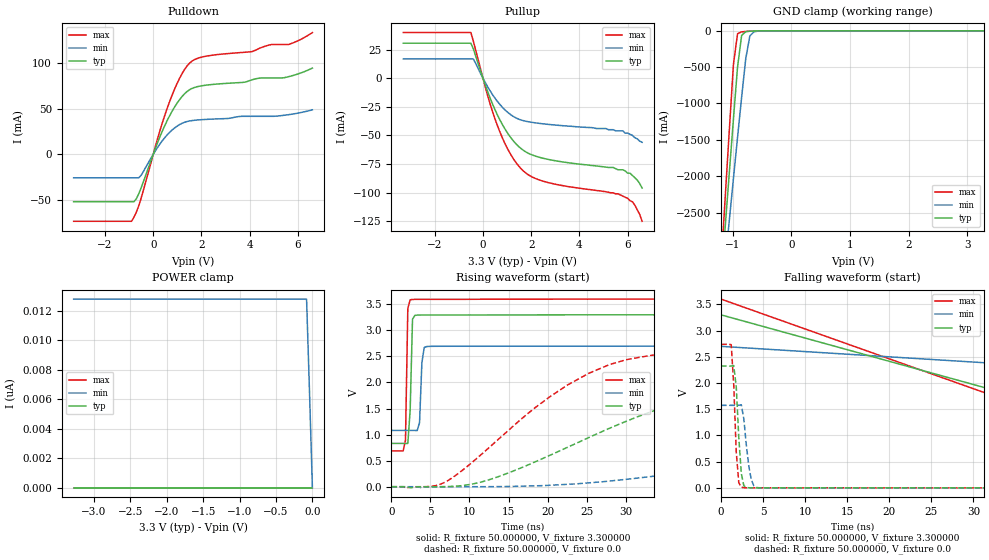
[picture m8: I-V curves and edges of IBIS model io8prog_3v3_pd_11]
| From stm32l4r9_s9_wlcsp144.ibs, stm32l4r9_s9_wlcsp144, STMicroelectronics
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|   Model io8prog_3v3_pd_11
[Model]  io8prog_3v3_pd_11
Model_type I/O
Polarity   Non-Inverting
Enable   Active-Low
Vinl =   0.990000V
Vinh =   2.310000V
Vmeas =  1.650000V
Cref =   100.000000nF
Rref =   1.000000k
Vref =   3.300000V
C_comp   2.267200pF   2.233100pF   2.322300pF
[Temperature Range]   25.000000   0.125000k   -40.000000
[Pullup Reference]   3.300000V   2.700000V   3.600000V
[Pulldown Reference]   0.0V   0.0V   0.0V
[POWER Clamp Reference]   3.300000V   2.700000V   3.600000V
[GND Clamp Reference]   0.0V   0.0V   0.0V
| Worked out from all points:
|   slope of the pulldown table from 0 to 0.495 V, typ, clamps not added: 15.3 ohm
|   slope of the pullup table from 0 to 0.495 V, typ, clamps not added: 18.1 ohm
|   GND clamp passes 1 mA (typ) near -0.58 V on its own axis
|   rising waveform, R_fixture 50.000000, V_fixture 3.300000: 20-80 % time 299ps typ, 253ps min, 207ps max; typ from 0.831 V to 3.3 V
|   rising waveform, R_fixture 50.000000, V_fixture 0.0: 20-80 % time 24.3ns typ, 50.8ns min, 14.5ns max; typ from 0 V to 2.32 V
|   falling waveform, R_fixture 50.000000, V_fixture 3.300000: 20-80 % time 33.4ns typ, 61.6ns min, 30.7ns max; typ from 3.3 V to 0.831 V
|   falling waveform, R_fixture 50.000000, V_fixture 0.0: 20-80 % time 498ps typ, 673ps min, 456ps max; typ from 2.32 V to 0 V
[Pulldown]
|Voltage   I(typ)   I(min)   I(max)
-3.3V     -51.86mA   -25.67mA   -73.32mA
-900mV    -51.86mA   -25.67mA   -73.32mA
-700mV    -48.68mA   -25.67mA   -63.27mA
-500mV    -36.68mA   -22.92mA   -47.9mA
200mV     14.09mA    8.363mA    18.97mA
700mV     43.2mA     24.54mA    59.15mA
1.2V      63.38mA    34mA       88.53mA
1.6V      72.01mA    36.89mA    101.8mA
4.1V      81.58mA    41.61mA    112.4mA
4.9V      83.61mA    41.61mA    120.1mA
5.6V      84.89mA    43.33mA    120.1mA
6.6V      94.39mA    48.68mA    133.3mA
[Pullup]
|Voltage   I(typ)   I(min)   I(max)
-3.3V     30.51mA    16.73mA    39.79mA
-500mV    30.51mA    16.73mA    39.79mA
-400mV    25.73mA    16.73mA    32.44mA
200mV     -11.99mA   -7.69mA    -15.6mA
500mV     -27.53mA   -17.49mA   -35.6mA
1V        -47.29mA   -29.38mA   -60.81mA
1.5V      -60.05mA   -35.95mA   -77.15mA
1.9V      -65.77mA   -38.13mA   -84.64mA
2.6V      -70.47mA   -40.14mA   -90.6mA
5.6V      -80mA      -46mA      -101mA
6.2V      -85mA      -50mA      -108mA
6.6V      -96mA      -56mA      -125mA
[GND_clamp]
|Voltage   I(typ)   I(min)   I(max)
-3.3V     -9.456A    -9.706A    -9.779A
-1.2V     -3.441A    -3.76A     -3.218A
-1.13V    -2.694A    -3.182A    -2.288A
-1.06V    -1.951A    -2.607A    -1.365A
-990mV    -1.216A    -2.035A    -464.9mA
-920mV    -500mA     -1.468A    -40.16mA
-850mV    -63.52mA   -913mA     -13.8mA
-780mV    -11.85mA   -384.3mA   -8.868mA
-710mV    -4.793mA   -70.28mA   -5.239mA
-640mV    -2.262mA   -14.31mA   -2.457mA
-430mV    -37.93uA   -161.8uA   -20.28uA
3.28V     87.11uA    89uA       71.58uA
[POWER_clamp]
|Voltage   I(typ)   I(min)   I(max)
-3.28V    0A         12.77nA    0A
-80mV     0A         12.77nA    0A
-40mV     0A         6.549nA    0A
0V        0A         0A         0A
[Ramp]
| variable   typ   min   max
dV/dt_r  1.39404/24.31899n   0.94416/54.54979n   1.64262/14.56547n
dV/dt_f  1.48081/21.07455n   0.97074/44.50667n   1.74729/13.65241n
R_load = 50.000000
[Rising Waveform]
R_fixture= 50.000000
V_fixture= 3.300000
V_fixture_min= 2.700000
V_fixture_max= 3.600000
|time   V(typ)   V(min)   V(max)
0s        830.9mV    1.081V     687.1mV
1.502ns   830.9mV    1.081V     686.2mV
1.802ns   830.5mV    1.081V     890.1mV
2.102ns   830.7mV    1.081V     3.419V
2.402ns   1.471V     1.081V     3.586V
2.703ns   3.213V     1.08V      3.593V
3.604ns   3.294V     1.23V      3.595V
3.904ns   3.294V     2.381V     3.595V
4.505ns   3.295V     2.689V     3.595V
149.5ns   3.299V     2.699V     3.599V
[Rising Waveform]
R_fixture= 50.000000
V_fixture= 0.0
V_fixture_min= 0.0
V_fixture_max= 0.0
|time   V(typ)   V(min)   V(max)
0s        2.475nV    39.58nV    2.334nV
6.607ns   913.9uV    -160.3uV   68.16mV
12.61ns   138.3mV    1.175mV    764.4mV
22.52ns   754mV      45.42mV    1.948V
27.93ns   1.121V     108.7mV    2.343V
33.33ns   1.442V     197mV      2.522V
46.85ns   1.993V     475.1mV    2.669V
64.56ns   2.218V     853.9mV    2.719V
98.5ns    2.306V     1.351V     2.736V
149.5ns   2.323V     1.574V     2.738V
[Falling Waveform]
R_fixture= 50.000000
V_fixture= 3.300000
V_fixture_min= 2.700000
V_fixture_max= 3.600000
|time   V(typ)   V(min)   V(max)
0s        3.299V     2.699V     3.599V
50.05ns   1.083V     2.199V     749.3mV
100.1ns   858.2mV    1.294V     691.5mV
150.2ns   835.9mV    1.141V     687.6mV
200.2ns   831.9mV    1.101V     687.1mV
300.3ns   830.9mV    1.083V     687.1mV
4.955us   830.9mV    1.081V     687.1mV
[Falling Waveform]
R_fixture= 50.000000
V_fixture= 0.0
V_fixture_min= 0.0
V_fixture_max= 0.0
|time   V(typ)   V(min)   V(max)
0s        2.323V     1.574V     2.738V
1.201ns   2.323V     1.574V     2.731V
1.502ns   2.331V     1.574V     1.966V
1.802ns   1.921V     1.574V     679.1mV
2.102ns   961.4mV    1.574V     95.31mV
2.402ns   274.6mV    1.584V     13.42mV
2.703ns   41.01mV    1.312V     2.637mV
3.604ns   774.4uV    146.2mV    498.7uV
4.505ns   320.9uV    2.033mV    459.9uV
149.5ns   2.475nV    39.58nV    2.334nV
